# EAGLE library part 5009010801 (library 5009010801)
Conn Micro SD Card HDR 8 POS 1.1mm Solder RA SMD 0.5A/Contact T/R Source: Datasheet
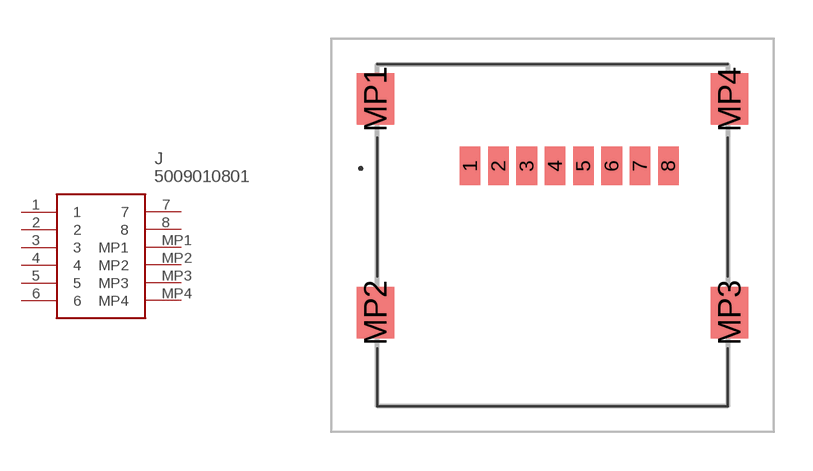
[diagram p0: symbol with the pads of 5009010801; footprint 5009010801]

Designator prefix J

## 5009010801 (Arrow_Part_Number: 5009010801; Arrow_Price-Stock: https://www.arrow.com/en/products/5009010801/molex?region=europe; Description: Conn Micro SD Card HDR 8 POS 1.1mm Solder RA SMD 0.5A/Contact T/R; Height: 2.13mm; Manufacturer_Name: Molex; Manufacturer_Part_Number: 5009010801)  [5009010801]
1  1
2  2
3  3
4  4
5  5
6  6
7  7
8  8
MP1  MP1
MP2  MP2
MP3  MP3
MP4  MP4

## Footprint 5009010801 (pad centres in mm)
5009010801-2
smd 0.8 x 1.5: 1 -3.2,2.7; 2 -2.1,2.7; 3 -1,2.7; 4 0.1,2.7; 5 1.2,2.7; 6 2.3,2.7; 7 3.4,2.7; 8 4.5,2.7
smd 1.45 x 2: MP1 -6.875,5.3; MP2 -6.875,-3; MP3 6.875,-3; MP4 6.875,5.3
